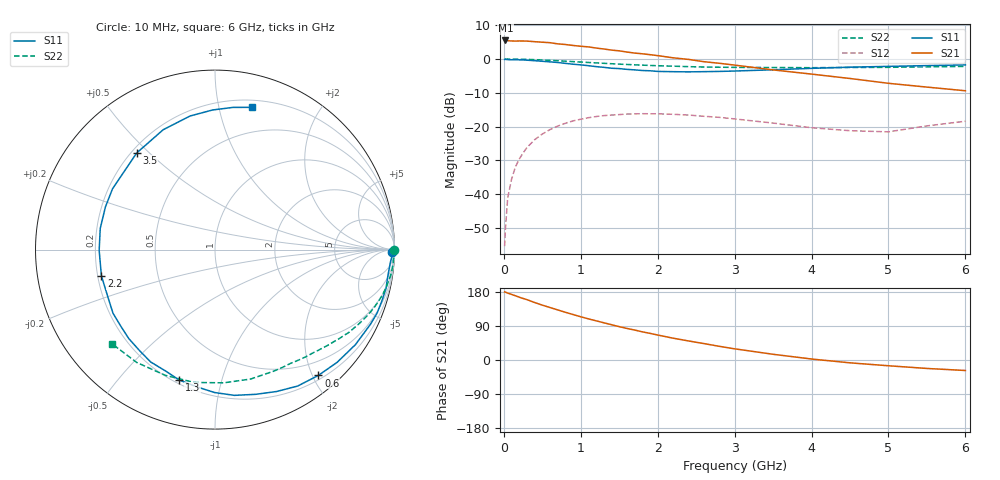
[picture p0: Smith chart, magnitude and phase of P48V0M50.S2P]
! SIEMENS Small Signal Semiconductors
! BFP182
! Si NPN RF Bipolar Junction Transistor in SOT143
! VCE = 8 V  IC = 0.5 mA
! Common Emitter S-Parameters:  March  1996
# GHz  S  MA  R  50
!  f  S11  S21  S12  S22
! GHz  MAG  ANG  MAG  ANG  MAG  ANG  MAG  ANG
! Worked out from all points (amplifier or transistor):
!   36 points, 10 MHz to 6 GHz, reference 50 ohm
!   highest |S21| = 5.5 dB at 20 MHz (marker M1)
!   |S21| within 3 dB of that: start of sweep to 1.466 GHz
!   unconditionally stable (mu >= 1): 2.95 GHz to end of sweep
!   at 250 MHz: K = 0.09, MSG = 16.6 dB, |S12| = -27.8 dB
!   at 1.4 GHz: K = 0.49, MSG = 9.6 dB, |S12| = -16.6 dB
!   at 6 GHz: K = 1.22, MAG = 1.7 dB, |S12| = -18.4 dB
!   S11 on the Smith chart (normalised r, x): 10 MHz: 71, -65; 600 MHz: 0.26, -2.09; 1.3 GHz: 0.22, -0.74; 2.2 GHz: 0.22, -0.11; 3.5 GHz: 0.22, +0.46; 6 GHz: 0.26, +1.26
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0.01  0.9849 -0.8  1.864 179.7  0.0017 87.2  0.9986 -0.2
0.02  0.9886 -1.6  1.882 179.2  0.003 86.9  0.9928 -0.5
0.05  0.9798 -4.1  1.865 176.5  0.0088 88.2  0.9989 -1.5
0.1  0.9742 -8.6  1.851 173.1  0.0166 83.3  0.9955 -3.1
0.15  0.9772 -13.0  1.842 169.6  0.0252 81.0  0.996 -4.7
0.3  0.9611 -25.6  1.841 159.3  0.0489 73.2  0.9865 -9.1
0.4  0.9447 -34.1  1.805 151.7  0.0639 67.8  0.9781 -12.0
0.6  0.9072 -50.6  1.744 138.5  0.0904 57.0  0.9552 -17.6
0.8  0.862 -66.5  1.64 125.9  0.1119 47.2  0.9287 -22.8
1.1  0.7963 -90.2  1.512 108.5  0.1354 34.3  0.8887 -29.5
1.3  0.7533 -105.4  1.407 98.2  0.1454 26.4  0.8636 -33.6
1.5  0.7215 -119.8  1.321 88.0  0.1505 19.7  0.8396 -37.4
1.8  0.6761 -141.1  1.195 74.3  0.1551 10.8  0.8118 -42.5
2.2  0.6495 -167.0  1.042 57.6  0.152 0.6  0.7835 -49.5
2.4  0.6454 -179.6  0.987 50.3  0.1482 -3.8  0.7712 -53.1
2.8  0.6552 158.7  0.865 36.1  0.1371 -10.3  0.7562 -60.2
3.5  0.693 129.0  0.69 15.1  0.1127 -16.4  0.748 -74.6
4  0.7275 113.4  0.598 2.6  0.0962 -13.4  0.7439 -86.2
4.5  0.7571 100.6  0.515 -7.5  0.0869 -6.7  0.7491 -98.8
5  0.778 91.0  0.437 -15.2  0.0836 7.1  0.7533 -111.5
5.5  0.7986 82.8  0.384 -22.3  0.1024 14.3  0.7653 -124.8
6  0.8183 75.6  0.339 -27.7  0.12 15.7  0.7777 -137.6
